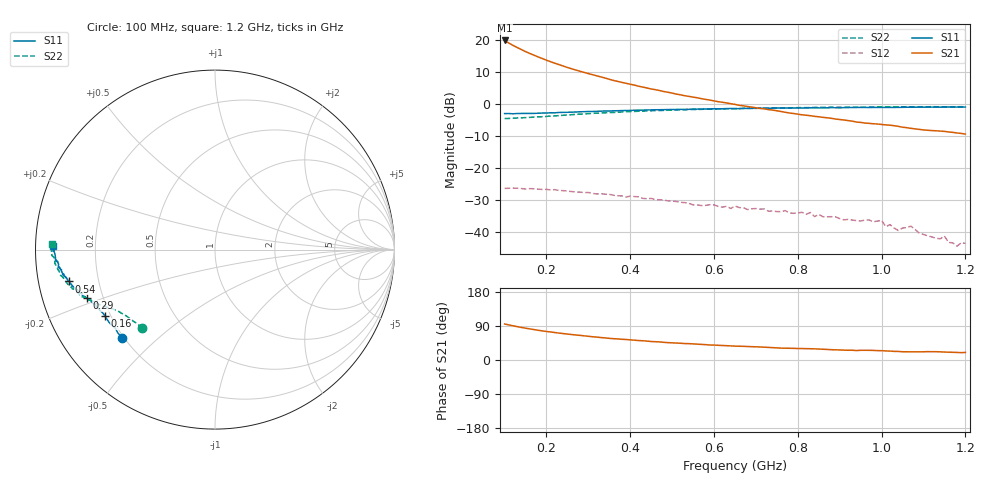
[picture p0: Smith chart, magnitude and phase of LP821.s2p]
! SCATTERING PARAMETERS :
!  POLYFET RF DEVICES
!  LP821/LQ821  /  L2C 1 Die
!  S PARAMETERS
!  VDS=12.5V, IDQ=100mA
# MHZ S MA R 50
! Freq=Mhz Mag[s11] Ang[s11] Mag[s21] Ang[s21] Mag[s12] Ang[s12] Mag[s22] Ang[s22]
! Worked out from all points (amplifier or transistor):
!   111 points, 100 MHz to 1.2 GHz, reference 50 ohm
!   highest |S21| = 20.0 dB at 100 MHz (marker M1)
!   |S21| within 3 dB of that: start of sweep to 142.3 MHz
!   unconditionally stable (mu >= 1): 659.9202 MHz to 660.1283 MHz; 678.2 MHz to 683.8 MHz; 722.4 MHz to end of sweep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
!   at 280 MHz: K = 0.33, MSG = 19.0 dB, |S12| = -27.6 dB
!   at 650 MHz: K = 0.84, MSG = 15.9 dB, |S12| = -31.9 dB
!   at 1.2 GHz: K = 6.35, MAG = 6.1 dB, |S12| = -43.6 dB
!   S11 on the Smith chart (normalised r, x): 100 MHz: 0.19, -0.39; 160 MHz: 0.18, -0.27; 290 MHz: 0.14, -0.18; 540 MHz: 0.09, -0.11; 1.2 GHz: 0.05, +0.01
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100  0.7125 -136.4  10 95.1  0.0477 4.5  0.5962 -132.7
110  0.7131 -139.4  9.117 92.6  0.04799 2.2  0.5973 -135.2
120  0.7072 -141.8  8.372 90.3  0.04823 -0.3  0.6017 -137.7
140  0.716 -145.8  7.203 85.9  0.04742 -5.0  0.6111 -141.3
160  0.7161 -149.0  6.251 82.1  0.04739 -8.4  0.6213 -144.2
190  0.7266 -152.4  5.204 76.9  0.04596 -12.8  0.6363 -147.1
220  0.732 -155.2  4.392 72.4  0.04564 -16.3  0.6549 -149.5
250  0.7463 -157.3  3.764 68.4  0.04343 -20.5  0.6763 -151.5
290  0.7628 -159.3  3.151 63.7  0.04102 -23.0  0.703 -153.7
360  0.787 -162.0  2.358 56.3  0.03723 -29.6  0.7413 -157.3
420  0.8044 -164.2  1.913 51.3  0.03521 -34.1  0.7758 -160.0
470  0.8194 -165.7  1.637 47.7  0.03174 -37.9  0.7968 -162.0
540  0.8315 -167.7  1.327 43.2  0.02776 -42.2  0.8246 -164.6
650  0.8532 -170.6  0.9933 36.6  0.02528 -41.3  0.852 -168.2
840  0.8774 -174.3  0.6447 29.4  0.01724 -52.5  0.8891 -173.9
1020  0.8907 -177.5  0.468 23.5  0.01288 -46.9  0.9101 -178.4
1040  0.8918 -178.4  0.4491 22.6  0.01044 -48.3  0.9102 -179.3
1070  0.8973 -179.3  0.4177 21.5  0.01218 -55.8  0.9112 -179.9
1110  0.9005 -179.6  0.3899 22.1  0.0086 -59.4  0.9107 179.3
1150  0.9006 -179.7  0.3741 21.0  0.00852 -49.0  0.9108 178.5
1180  0.9014 179.6  0.3538 19.9  0.00592 -40.3  0.9111 178.3
1200  0.9013 178.6  0.3399 20.0  0.00657 -30.6  0.9108 178.1
